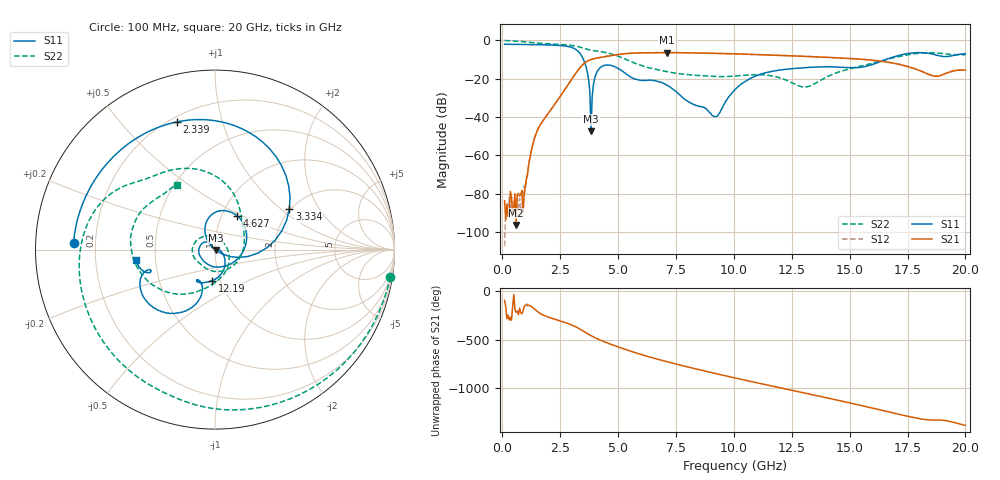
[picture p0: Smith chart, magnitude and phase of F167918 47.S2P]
!  2-Port S-parameters saved by WinCal
! VAR MeasName=S-Parameters (CALIBRATED_DATA) read from VNA (N5242A)
! VAR MeasDate=2016-11-22 10:27:04
! VAR NAME=F167918 47
! VAR FILENAME=F167918 47.S2P
! VAR DATE=2016-11-22 10:27:04
! VAR PHYS_PORTS=1,2
# Hz S DB R 50
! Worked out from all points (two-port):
!   401 points, 100 MHz to 20 GHz, reference 50 ohm
!   highest |S21| = -6.40 dB at 7.115 GHz (marker M1); lowest = -96.2 dB at 597.5 MHz (marker M2)
!   |S21| within 3 dB of the highest: 4.022 GHz to 14.81 GHz (10.79 GHz wide, 115 % of centre)
!   lowest |S11| = -47.3 dB at 3.831 GHz (marker M3), VSWR 1.01, Z = 50.4 - j0.249 ohm
!   |S11| at or under -10 dB: 3.505 GHz to 16.57 GHz (13.07 GHz wide, 130 % of centre)
!   |S22| runs from -24.3 to -0.1 dB; largest |S21 - S12| = 0.0049
!   S11 on the Smith chart (normalised r, x): 100 MHz: 0.12, +0.02; 2.339 GHz: 0.23, +0.72; 3.334 GHz: 1.97, +1.15; 4.627 GHz: 1.18, +0.47; 12.19 GHz: 0.92, -0.33; 20 GHz: 0.39, -0.06
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1e8  -2.07 177.3  -83.57 -95.0  -107.22 46.8  -0.10 -8.8
5.975e8  -2.13 164.0  -96.23 141.6  -84.17 144.3  -0.45 -48.6
9.4575e8  -2.19 154.6  -80.77 -158.2  -75.97 -163.4  -0.78 -74.2
1.493e9  -2.30 138.5  -47.47 154.2  -47.48 154.6  -1.45 -109.3
2.33875e9  -2.59 106.7  -31.99 64.6  -31.98 64.4  -2.07 -154.7
3.33375e9  -6.52 28.7  -14.58 -29.1  -14.59 -29.0  -3.49 153.9
3.43325e9  -8.25 15.7  -13.20 -43.1  -13.20 -42.9  -3.84 149.0
3.83125e9  -47.31 -34.9  -10.02 -99.9  -10.00 -100.0  -5.18 134.4
4.12975e9  -15.71 106.7  -9.15 -135.2  -9.14 -135.5  -5.71 123.7
4.62725e9  -12.95 57.0  -8.12 176.9  -8.14 176.7  -6.84 101.5
5.672e9  -19.95 -74.1  -6.65 90.0  -6.65 89.9  -11.68 57.7
6.7665e9  -21.55 161.2  -6.42 13.2  -6.42 13.1  -15.51 13.8
7.11475e9  -23.41 141.5  -6.40 -9.0  -6.43 -9.0  -16.35 -6.4
8.1595e9  -32.87 139.1  -6.55 -72.0  -6.56 -72.1  -18.07 -74.8
9.20425e9  -39.75 76.0  -6.83 -130.8  -6.83 -130.9  -18.81 -122.8
1.005e10  -25.67 -29.9  -7.07 -176.7  -7.09 -176.5  -18.66 -144.4
1.218925e10  -15.21 -94.9  -7.96 72.0  -7.94 72.0  -20.45 129.0
1.338325e10  -14.07 -111.4  -8.55 10.6  -8.49 10.6  -23.30 4.8
1.507475e10  -14.30 -119.0  -9.55 -77.3  -9.52 -77.7  -14.66 -90.4
1.67165e10  -9.41 -111.0  -11.53 -168.4  -11.50 -168.4  -9.62 -131.6
1.825875e10  -6.56 -151.8  -16.96 114.3  -16.87 113.7  -6.52 175.1
2e10  -7.03 -172.5  -15.53 53.0  -15.47 52.2  -7.52 120.6
